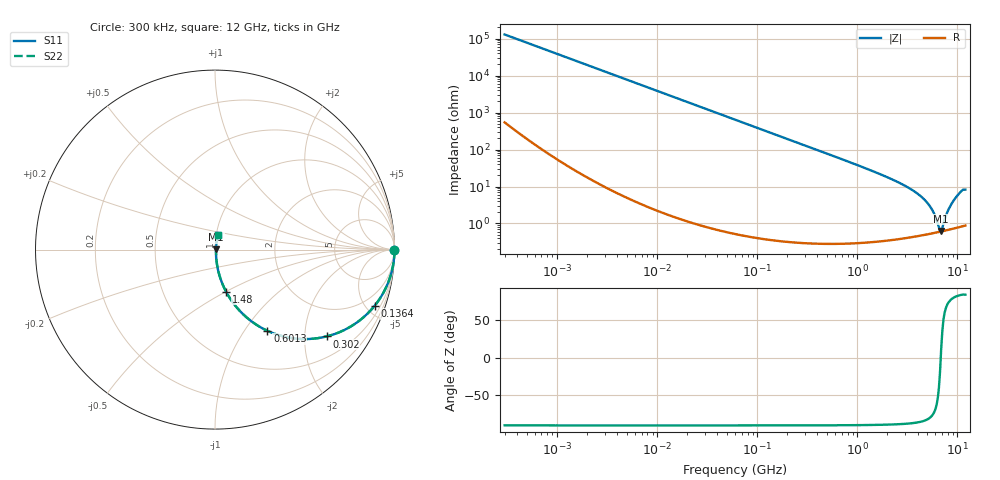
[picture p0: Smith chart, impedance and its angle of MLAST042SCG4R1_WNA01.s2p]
! MLAST042SCG4R1_WNA01  S-PARAMETER MODEL  ( General Type )
! Model Generated by TAIYO YUDEN Corporation (http://www.ty-top.com)
! Version 1.0
! TAIYO YUDEN Control No. 150820
! Copyright(c) 2015 TAIYO YUDEN CO.,LTD. All Rights Reserved.
! Product Description (link to TY-COMPAS)
! https://ds.yuden.co.jp/TYCOMPAS/or/detail?pn=MLAST042SCG4R1BWNA01&u=M
! Products Name : Multilayer Ceramic Capacitors
! Characteristics :
!  Capacitance : 4.1 pF , Rated Voltage : 25V , TCC : CG / C0G
!  Case Size : 0.4 x 0.2 / 0.016 x 0.008 [mm/inch] , Thickness : 0.2 / 0.008 [mm/inch]
!  (Conditions: Temperature = 25 degC , DC Bias Current/Voltage = 0A / 0V)
! External Node Assignments :
!  1  o---| |---o  2
! GND o---------o GND
! Frequency Range : 0.3MHz  -  12000MHz  [ 401 STEP ]
# MHz S RI R 50
! Freq[MHz].  S11 Real  S11 Imag  S21 Real  S21 Imag  S12 Real  S12 Imag  S22 Real  S22 Imag
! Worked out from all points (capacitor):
!   401 points, 300 kHz to 12 GHz, reference 50 ohm
!   read as one part in series: C = 4.1 pF near 316.3 kHz
!   lowest |Z| = 622 mohm at 6.88 GHz (marker M1)
!   series resonance near 6.808 GHz, so ESL is about 130 pH
!   S11 on the Smith chart (normalised r, x): 300 kHz: open; 136.4 MHz: 1.01, -5.69; 302 MHz: 1.01, -2.57; 601.3 MHz: 1.01, -1.28; 1.48 GHz: 1.01, -0.50; 12 GHz: 1.02, +0.16
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0.3  1 -0.000773  3.84e-06 0.000773  3.84e-06 0.000773  1 -0.000773
1.769972  1 -0.00456  2.52e-05 0.00456  2.52e-05 0.00456  1 -0.00456
10.44266  0.9993 -0.0269  0.000739 0.0269  0.000739 0.0269  0.9993 -0.0269
60  0.9765 -0.151  0.0235 0.151  0.0235 0.151  0.9765 -0.151
136.3989  0.8897 -0.3127  0.1103 0.3127  0.1103 0.3127  0.8897 -0.3127
301.9711  0.6217 -0.4838  0.3783 0.4838  0.3783 0.4838  0.6217 -0.4838
353.9943  0.5444 -0.4967  0.4556 0.4967  0.4556 0.4967  0.5444 -0.4967
601.3112  0.2917 -0.4524  0.7083 0.4524  0.7083 0.4524  0.2917 -0.4524
918.7169  0.1485 -0.3522  0.8515 0.3522  0.8515 0.3522  0.1485 -0.3522
1480.043  0.0614 -0.2338  0.9386 0.2338  0.9386 0.2338  0.0614 -0.2338
2088.533  0.0308 -0.1626  0.9692 0.1626  0.9692 0.1626  0.0308 -0.1626
3276.641  0.0123 -0.0896  0.9877 0.0896  0.9877 0.0896  0.0123 -0.0896
4502.883  0.0071 -0.048  0.9929 0.048  0.9929 0.048  0.0071 -0.048
5420.343  0.00595 -0.026  0.994 0.026  0.994 0.026  0.00595 -0.026
5868.704  0.0058 -0.0169  0.9942 0.0169  0.9942 0.0169  0.0058 -0.0169
6524.734  0.00588 -0.00492  0.9941 0.00492  0.9941 0.00492  0.00588 -0.00492
6879.757  0.00604 0.0013  0.994 -0.0013  0.994 -0.0013  0.00604 0.0013
7064.448  0.00616 0.00439  0.9938 -0.00439  0.9938 -0.00439  0.00616 0.00439
8064.993  0.00713 0.0215  0.9929 -0.0215  0.9929 -0.0215  0.00713 0.0215
8966.534  0.00852 0.0371  0.9915 -0.0371  0.9915 -0.0371  0.00852 0.0371
10793.46  0.0131 0.0703  0.9869 -0.0703  0.9869 -0.0703  0.0131 0.0703
12000  0.0152 0.0798  0.9848 -0.0798  0.9848 -0.0798  0.0152 0.0798
